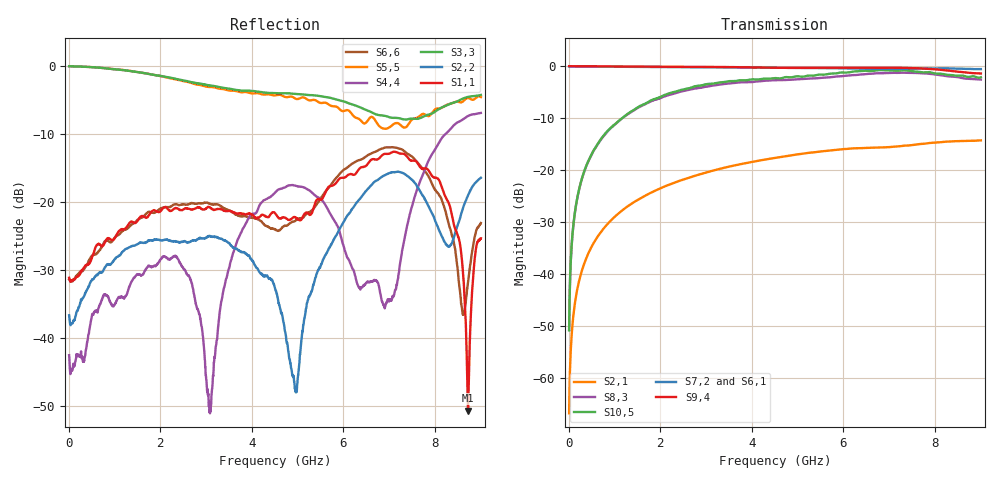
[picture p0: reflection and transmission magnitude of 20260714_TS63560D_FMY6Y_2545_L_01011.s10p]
# GHz S DB R 50
! CMT, SN0916, 25263762, 26.7.0
! Date: 15.07.2026 13:39:02
! Data: Format
! Freq S1.1:dB/Ang S1.2:dB/Ang S1.3:dB/Ang S1.4:dB/Ang S1.5:dB/Ang S1.6:dB/Ang S1.7:dB/Ang S1.8:dB/Ang S1.9:dB/Ang S1.10:dB/Ang
!  S2.1:dB/Ang S2.2:dB/Ang S2.3:dB/Ang S2.4:dB/Ang S2.5:dB/Ang S2.6:dB/Ang S2.7:dB/Ang S2.8:dB/Ang S2.9:dB/Ang S2.10:dB/Ang
!  S3.1:dB/Ang S3.2:dB/Ang S3.3:dB/Ang S3.4:dB/Ang S3.5:dB/Ang S3.6:dB/Ang S3.7:dB/Ang S3.8:dB/Ang S3.9:dB/Ang S3.10:dB/Ang
!  S4.1:dB/Ang S4.2:dB/Ang S4.3:dB/Ang S4.4:dB/Ang S4.5:dB/Ang S4.6:dB/Ang S4.7:dB/Ang S4.8:dB/Ang S4.9:dB/Ang S4.10:dB/Ang
!  S5.1:dB/Ang S5.2:dB/Ang S5.3:dB/Ang S5.4:dB/Ang S5.5:dB/Ang S5.6:dB/Ang S5.7:dB/Ang S5.8:dB/Ang S5.9:dB/Ang S5.10:dB/Ang
!  S6.1:dB/Ang S6.2:dB/Ang S6.3:dB/Ang S6.4:dB/Ang S6.5:dB/Ang S6.6:dB/Ang S6.7:dB/Ang S6.8:dB/Ang S6.9:dB/Ang S6.10:dB/Ang
!  S7.1:dB/Ang S7.2:dB/Ang S7.3:dB/Ang S7.4:dB/Ang S7.5:dB/Ang S7.6:dB/Ang S7.7:dB/Ang S7.8:dB/Ang S7.9:dB/Ang S7.10:dB/Ang
!  S8.1:dB/Ang S8.2:dB/Ang S8.3:dB/Ang S8.4:dB/Ang S8.5:dB/Ang S8.6:dB/Ang S8.7:dB/Ang S8.8:dB/Ang S8.9:dB/Ang S8.10:dB/Ang
!  S9.1:dB/Ang S9.2:dB/Ang S9.3:dB/Ang S9.4:dB/Ang S9.5:dB/Ang S9.6:dB/Ang S9.7:dB/Ang S9.8:dB/Ang S9.9:dB/Ang S9.10:dB/Ang
!  S10.1:dB/Ang S10.2:dB/Ang S10.3:dB/Ang S10.4:dB/Ang S10.5:dB/Ang S10.6:dB/Ang S10.7:dB/Ang S10.8:dB/Ang S10.9:dB/Ang S10.10:dB/Ang
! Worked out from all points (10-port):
!   2001 points, 10 MHz to 9 GHz, reference 50 ohm
!   strongest paths, dB at 10 MHz, 2.257 GHz, 4.505 GHz, 6.753 GHz, 9 GHz:
!     S9,4: -0.1, -0.2, -0.4, -0.4, -1.5
!     S7,2: -0.1, -0.3, -0.4, -0.6, -0.6
!     S6,1: -0.2, -0.4, -0.5, -0.7, -0.6
!     S10,5: -50.8, -5.1, -2.4, -0.8, -2.2
!     S8,3: -50.7, -5.5, -2.8, -1.4, -2.6
!     S2,1: -66.7, -22.6, -17.7, -15.7, -14.3
!   lowest |S11| = -50.7 dB at 8.721 GHz (marker M1), VSWR 1.01, Z = 49.9 + j0.263 ohm
!   |S11| at or under -10 dB: start of sweep to end of sweep
